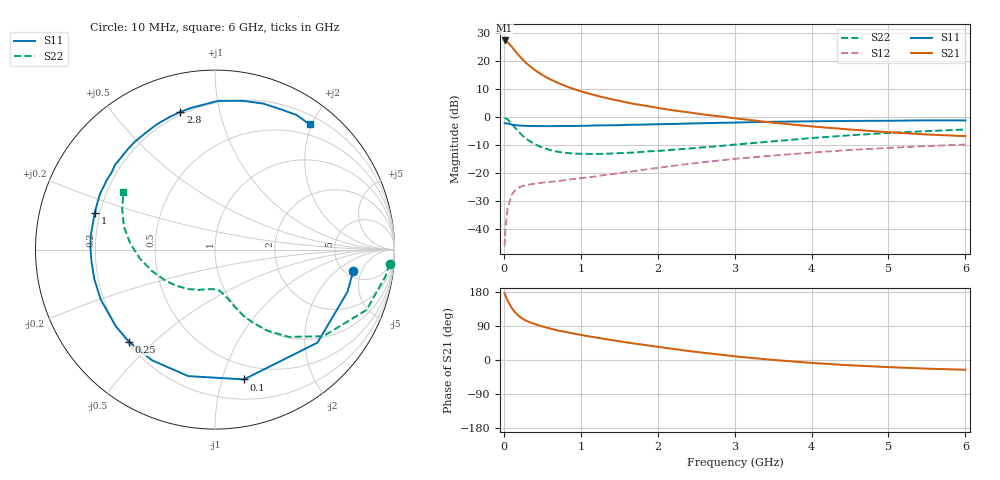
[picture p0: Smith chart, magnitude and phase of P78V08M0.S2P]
! SIEMENS Small Signal Semiconductors
! BFP196
! Si NPN RF Bipolar Junction Transistor in SOT143
! VCE = 8 V  IC = 8 mA
! Common Emitter S-Parameters:  May  1996
# GHz  S  MA  R  50
!  f  S11  S21  S12  S22
! GHz  MAG  ANG  MAG  ANG  MAG  ANG  MAG  ANG
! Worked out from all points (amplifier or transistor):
!   36 points, 10 MHz to 6 GHz, reference 50 ohm
!   highest |S21| = 27.4 dB at 10 MHz (marker M1)
!   |S21| within 3 dB of that: start of sweep to 124.7 MHz
!   unconditionally stable (mu >= 1): 999.4 MHz to 3.29 GHz
!   at 250 MHz: K = 0.33, MSG = 22.4 dB, |S12| = -24.5 dB
!   at 1.4 GHz: K = 1.14, MAG = 11.1 dB, |S12| = -20.4 dB
!   at 6 GHz: K = 0.96, MSG = 1.5 dB, |S12| = -9.7 dB
!   S11 on the Smith chart (normalised r, x): 10 MHz: 5.82, -3.58; 100 MHz: 0.37, -1.18; 250 MHz: 0.21, -0.42; 1 GHz: 0.18, +0.15; 2.8 GHz: 0.19, +0.76; 6 GHz: 0.33, +1.97
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0.01  0.7795 -8.9  23.34 176.0  0.005 87.0  0.9758 -4.7
0.02  0.7744 -17.8  22.77 169.9  0.0102 80.3  0.961 -9.0
0.05  0.7712 -42.2  21.48 156.7  0.024 69.9  0.9088 -21.7
0.1  0.741 -77.4  18.27 138.2  0.0411 54.3  0.7724 -38.7
0.15  0.7205 -101.9  14.9 124.6  0.0506 44.2  0.6355 -49.9
0.2  0.7094 -119.6  12.44 115.2  0.0561 38.4  0.5365 -57.2
0.25  0.7026 -132.9  10.44 107.9  0.0594 34.6  0.4574 -62.6
0.3  0.6984 -142.4  8.98 102.7  0.0618 32.4  0.404 -66.6
0.4  0.6948 -156.4  6.97 94.9  0.0652 30.4  0.3303 -71.4
0.5  0.6922 -166.4  5.643 88.5  0.0677 29.7  0.2863 -74.9
0.6  0.6915 -174.5  4.755 83.1  0.0703 30.4  0.2595 -78.3
0.7  0.6944 178.7  4.11 78.1  0.0722 31.1  0.2421 -81.1
0.8  0.6966 173.4  3.601 74.1  0.0756 32.3  0.2312 -83.7
1  0.7007 162.9  2.9 66.3  0.0817 34.7  0.2222 -88.4
1.1  0.7048 158.6  2.648 62.6  0.0846 36.2  0.2212 -91.3
1.6  0.7305 139.7  1.822 46.3  0.1051 40.3  0.2314 -105.8
2.2  0.7562 120.8  1.323 29.3  0.1354 40.9  0.2626 -122.7
2.8  0.7916 104.1  1.036 14.5  0.1686 38.0  0.3052 -141.3
3.5  0.8289 88.8  0.798 0.2  0.2069 31.7  0.3707 -161.2
4.5  0.8568 71.7  0.602 -13.9  0.2597 21.3  0.475 175.5
5.5  0.8771 58.7  0.491 -22.8  0.3053 9.7  0.5644 156.4
6  0.8741 52.9  0.459 -25.8  0.3257 3.5  0.6022 147.9
